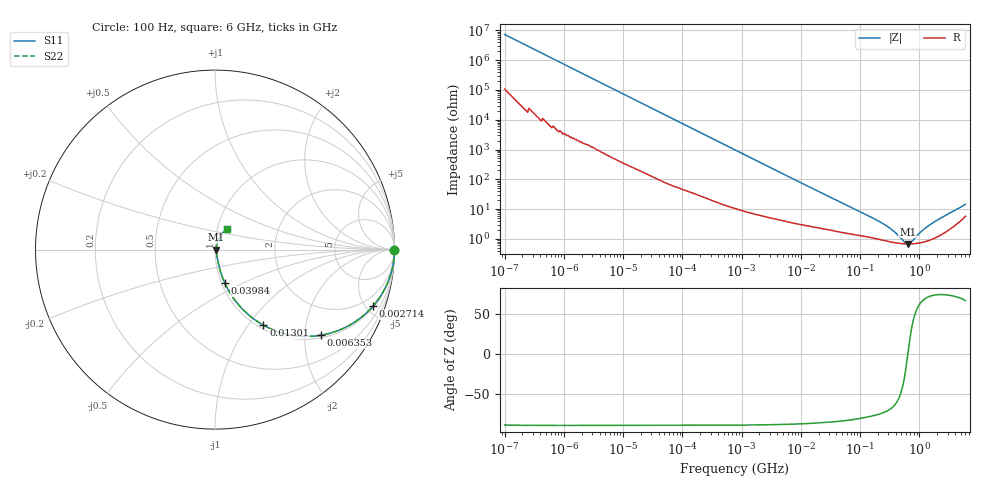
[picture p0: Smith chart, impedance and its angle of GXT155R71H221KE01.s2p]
!Murata Part Number: GXT155R71H221KE01
!These Parameters are Measured in Series Mode Connection
!Data Generated on Jan 08, 2026
!  o--ll--o
!Port1  Port2
!  o------o
!Operation Temp=25[degC], DC Bias Voltage=0[V]
!Freq. Start=100[Hz] Stop=6[GHz] 401[Steps]
# Hz S RI R 50
!Freq.(Hz) S11(Real) S11(Imag) S21(Real) S21(Imag) S12(Real) S12(Imag) S22(Real) S22(Imag)
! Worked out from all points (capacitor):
!   401 points, 100 Hz to 6 GHz, reference 50 ohm
!   read as one part in series: C = 218 pF near 109 Hz
!   lowest |Z| = 677 mohm at 639.6 MHz (marker M1)
!   series resonance near 641.5 MHz, so ESL is about 280 pH
!   S11 on the Smith chart (normalised r, x): 100 Hz: open; 2.714 MHz: 1.11, -5.57; 6.353 MHz: 1.07, -2.40; 13.01 MHz: 1.05, -1.19; 39.84 MHz: 1.04, -0.40; 6 GHz: 1.11, +0.27
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100  1 -1.37e-05  2e-07 1.37e-05  2e-07 1.37e-05  1 -1.37e-05
717  1 -9.78e-05  5e-07 9.78e-05  5e-07 9.78e-05  1 -9.78e-05
2008  1 -0.000273  1.4e-06 0.000273  1.4e-06 0.000273  1 -0.000273
40335  0.9999 -0.00544  5.77e-05 0.00544  5.77e-05 0.00544  0.9999 -0.00544
241822  0.9987 -0.0323  0.0013 0.0323  0.0013 0.0323  0.9987 -0.0323
774597  0.9884 -0.1019  0.0116 0.1019  0.0116 0.1019  0.9884 -0.1019
1585629  0.9549 -0.2003  0.0451 0.2003  0.0451 0.2003  0.9549 -0.2003
2713602  0.8813 -0.3139  0.1187 0.3139  0.1187 0.3139  0.8813 -0.3139
4060267  0.7724 -0.4076  0.2276 0.4076  0.2276 0.4076  0.7724 -0.4076
6353432  0.5882 -0.4774  0.4118 0.4774  0.4118 0.4774  0.5882 -0.4774
1.300572e7  0.2697 -0.4212  0.7303 0.4212  0.7303 0.4212  0.2697 -0.4212
1.555665e7  0.2106 -0.3826  0.7894 0.3826  0.7894 0.3826  0.2106 -0.3826
2.434276e7  0.1093 -0.2799  0.8907 0.2799  0.8907 0.2799  0.1093 -0.2799
3.983537e7  0.0537 -0.1849  0.9463 0.1849  0.9463 0.1849  0.0537 -0.1849
1.669249e8  0.0128 -0.047  0.9872 0.047  0.9872 0.047  0.0128 -0.047
3.124326e8  0.00847 -0.0218  0.9915 0.0218  0.9915 0.0218  0.00847 -0.0218
5.59173e8  0.0068 -0.00396  0.9932 0.00396  0.9932 0.00396  0.0068 -0.00396
6.395615e8  0.00672 -8.54e-05  0.9933 8.54e-05  0.9933 8.54e-05  0.00672 -8.54e-05
7.31507e8  0.00676 0.00381  0.9932 -0.00381  0.9932 -0.00381  0.00676 0.00381
1.094528e9  0.00772 0.0162  0.9923 -0.0162  0.9923 -0.0162  0.00772 0.0162
1.565993e9  0.0101 0.0292  0.9899 -0.0292  0.9899 -0.0292  0.0101 0.0292
6e9  0.069 0.1175  0.931 -0.1175  0.931 -0.1175  0.069 0.1175
